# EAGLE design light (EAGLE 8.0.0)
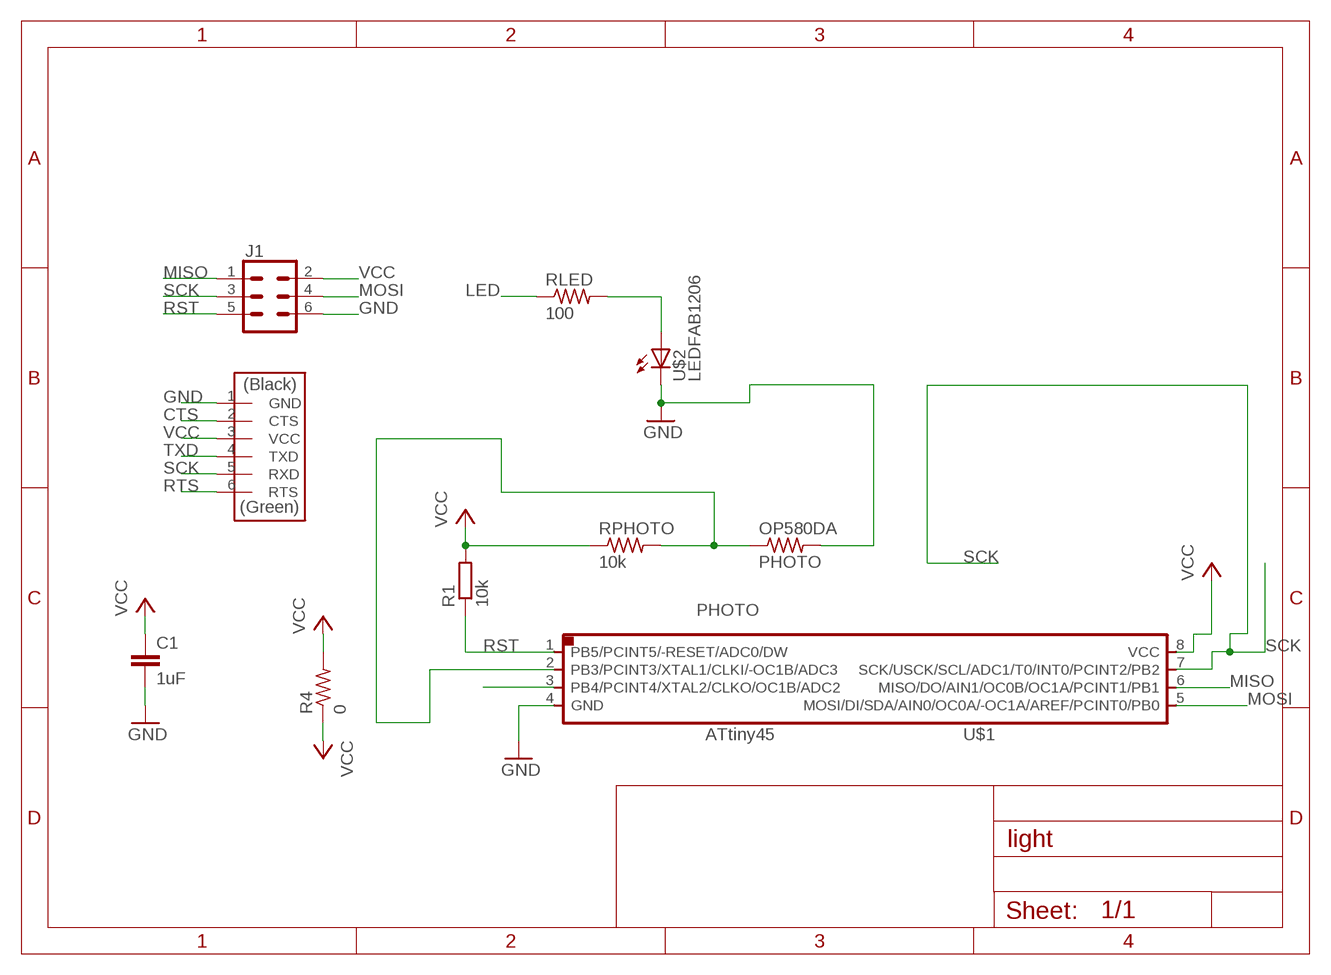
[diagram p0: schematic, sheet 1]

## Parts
C1  1uF  C-EUC1206  [C1206]
J1  CONN_03X2SMT  [2X3_SMT_POSTS]
J2  FTDI-SMD-HEADER  [1X06SMD]
OP580DA  PHOTO  RES-US1206  [R1206]
R1  10k  R-EU_M1206  [M1206]
R4  0  RES-US1206FAB  [R1206FAB]
RLED  100  RES-US1206  [R1206]
RPHOTO  10k  RES-US1206  [R1206]
U$1  ATTINY45SI  [SOIC8]
U$2  LEDFAB1206  [LED1206FAB]

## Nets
CTS: J2.2(CTS)
GND: C1.2 J1.6 J2.1(GND) OP580DA.2 U$1.4(GND) U$2.2(C)
LED: RLED.1 U$1.3(PB4/PCINT4/XTAL2/CLKO/OC1B/ADC2)
MISO: J1.1 U$1.6(MISO/DO/AIN1/OC0B/OC1A/PCINT1/PB1)
MOSI: J1.4 U$1.5(MOSI/DI/SDA/AIN0/OC0A/-OC1A/AREF/PCINT0/PB0)
N$1: RLED.2 U$2.1(A)
PHOTO: OP580DA.1 RPHOTO.2 U$1.2(PB3/PCINT3/XTAL1/CLKI/-OC1B/ADC3)
RST: J1.5 R1.1 U$1.1(PB5/PCINT5/-RESET/ADC0/DW)
RTS: J2.6(RTS)
SCK: J1.3 J2.5(RXD) U$1.7(SCK/USCK/SCL/ADC1/T0/INT0/PCINT2/PB2)
TXD: J2.4(TXD)
VCC: C1.1 J1.2 J2.3(VCC) R1.2 R4.1 R4.2 RPHOTO.1 U$1.8(VCC)

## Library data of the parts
C1 = rcl:C-EU: CAPACITOR, European symbol
J1 = SparkFun-Connectors:CONN_03X2: Multi connection point. Often used as Generic Header-pin footprint for 0.1 inch spaced/style header connections You can populate with any combo of single row headers, but if you'd like an exact match, check these: Header - 2x3 (Male, 0.1") (PRT-12807) Header - 2x3 (Female, 0.1") (PRT-13010) 2x3 Pin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; PROD_ID: CONN-11415
J2 = fab:FTDI-SMD-HEADER
OP580DA R4 RLED RPHOTO = fab:RES-US: Resistor (US Symbol)
R1 = rcl:R-EU_: RESISTOR, European symbol
U$1 = fab:ATTINY45
U$2 = fab:LED: LED

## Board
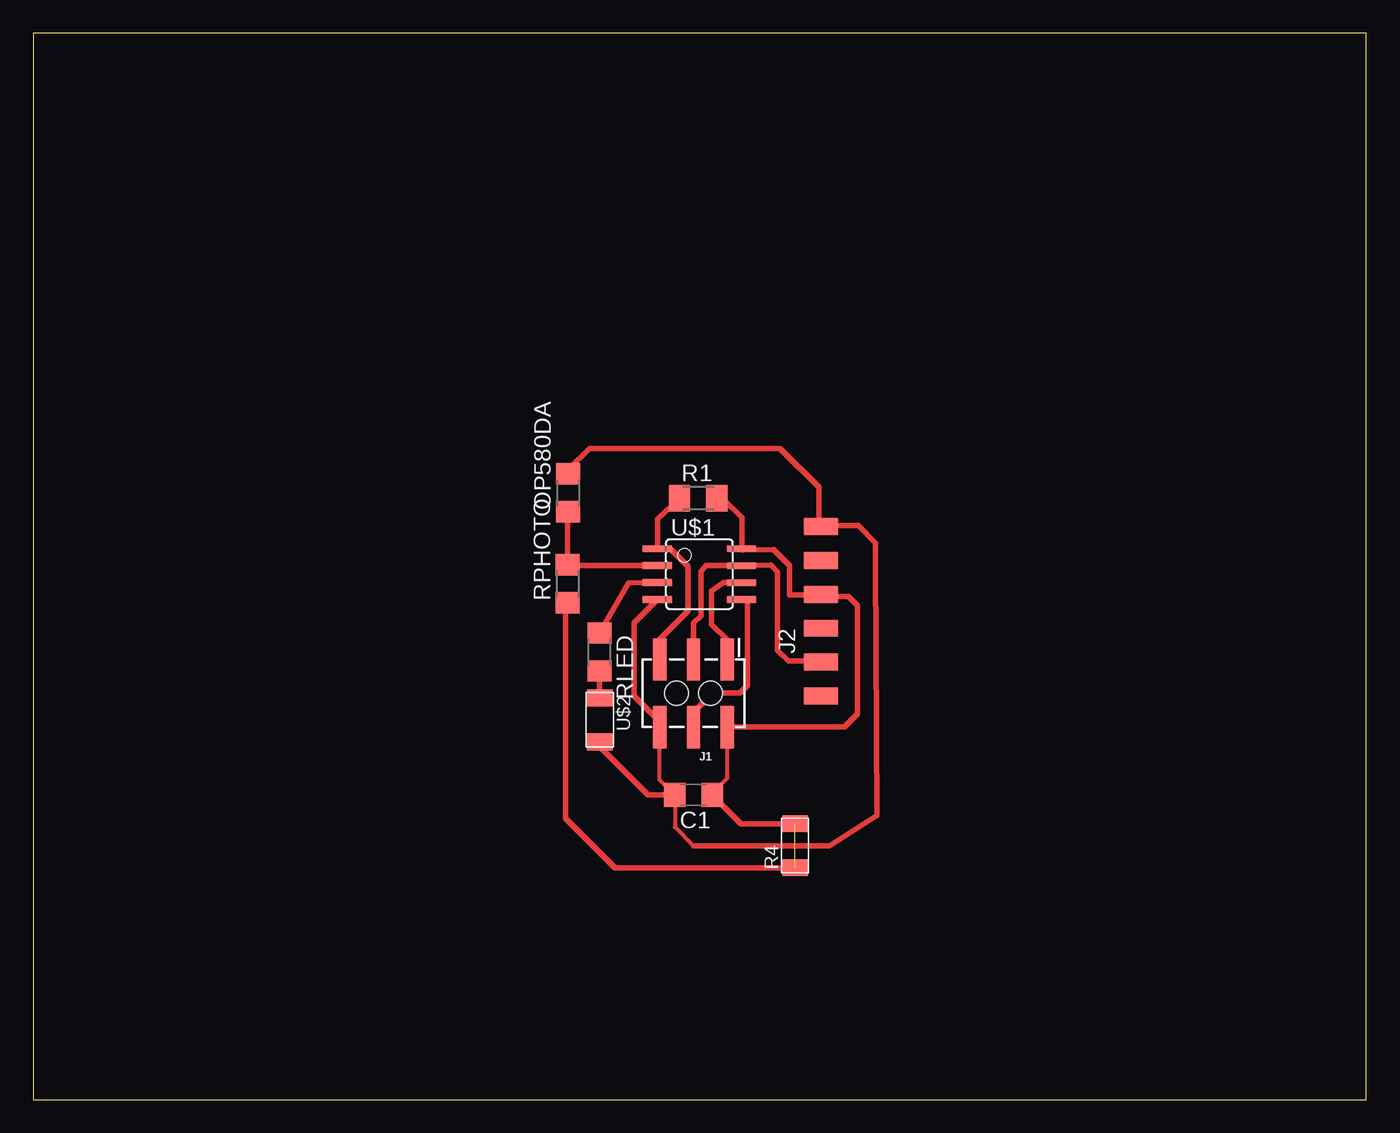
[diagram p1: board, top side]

Size 100 x 80 mm. Coordinates in mm from the lower left corner, seen from the top.
Outline: 0,0 100,0 100,80 0,80 0,0
Copper layers (1*16): Top 0.035mm / dielectric 1.5mm / Bottom 0.035mm
Design rules "default *": minimum track width 12mil, minimum drill 16mil, track to track 16mil, track to pad 16mil, pad to pad 16mil, via to via 16mil, smd to smd 16mil, copper to edge 16mil, drill to drill 16mil, minimum pad ring 10mil, minimum via ring 8mil, stop-mask expansion 4mil, vias tented up to drill 0mil, thermal gap 10mil

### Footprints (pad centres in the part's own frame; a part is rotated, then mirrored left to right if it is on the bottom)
C1206 = smd 1.6 x 1.8: 1 -1.4,0; 2 1.4,0
2X3_SMT_POSTS = smd 1 x 3.17: 1 -2.54,-2.54; 2 -2.54,2.54; 3 0,-2.54; 4 0,2.54; 5 2.54,-2.54; 6 2.54,2.54 | hole 1.8: -1.27,0; 1.27,0
1X06SMD = smd 2.54 x 1.27: 1 0,6.35; 2 0,3.81; 3 0,1.27; 4 0,-1.27; 5 0,-3.81; 6 0,-6.35
R1206 = smd 1.6 x 1.803: 1 -1.422,0; 2 1.422,0
M1206 = smd 1.6 x 2: 1 -1.4,0; 2 1.4,0
R1206FAB = smd 1.27 x 1.905: 1 -1.651,0; 2 1.651,0
SOIC8 = smd 0.5 x 2.2: 1 -1.905,-3.154; 2 -0.645,-3.154; 3 0.625,-3.154; 4 1.895,-3.154; 5 1.905,3.154; 6 0.635,3.154; 7 -0.635,3.154; 8 -1.905,3.154
LED1206FAB = smd 1.27 x 1.905: 1 -1.651,0; 2 1.651,0

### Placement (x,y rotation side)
C1  49.53,22.86 180 top
J1  49.53,30.48 180 top
J2  59.1,36.63 0 top
OP580DA  40.12,45.52 90 top
R1  49.89,45.1 0 top
R4  57.15,19.05 90 top
RLED  42.49,33.58 270 top
RPHOTO  40.09,38.7 90 top
U$1  49.97,39.42 270 top
U$2  42.5,28.49 270 top

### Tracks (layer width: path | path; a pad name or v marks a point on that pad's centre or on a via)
GND
  Top 0.305: J1.6 46.99,24 C1.2 48.13,20.45 49.53,19.05
  Top 0.406: J1.6 46.99,28.35 45.06,30.28 45.06,35.77 U$1.4 | 49.53,19.05 59.73,19.05 63.3,21.32 63.18,40.19 63.18,41.76 61.89,43.06 59.18,43.06 J2.1 58.92,43.16 58.92,45.94 56.03,48.84 45.02,48.84 45,48.85 41.72,48.85 40.12,47.26 OP580DA.2 | U$2.2 42.5,26.48 46.11,22.87 C1.2
LED
  Top 0.406: U$1.3 44.67,38.77 RLED.1
MISO
  Top 0.406: J1.1 52.07,34.47 50.9,35.64 50.9,38.16 51.79,38.78 53.14,38.78 U$1.6
MOSI
  Top 0.406: J1.4 49.53,29.06 50.99,30.51 53.02,30.51 53.59,31.08 53.59,36.97 | 53.59,37.35 53.59,36.97 | 53.59,37.35 53.72,37.48 53.59,37.35 | 53.59,36.97 53.59,37.35 | U$1.5 53.44,37.51 53.59,37.35
N$1
  Top 0.406: RLED.2 42.49,30.16 U$2.1
PHOTO
  Top 0.406: OP580DA.1 40.09,43.71 RPHOTO.2 40.15,40.06 U$1.2 46.19,40.11
RST
  Top 0.305: 46.99,34.29 J1.5
  Top 0.406: J1.5 46.99,34.53 49.12,36.66 49.11,40.01 47.81,41.31 47.13,41.29 | 47.13,41.29 46.3,41.26 | R1.1 46.82,43.56 U$1.1 47.09,41.32 47.13,41.29
SCK
  Top 0.406: J1.3 49.53,35.77 50.08,36.28 50.08,39.63 50.48,40.07 53.11,40.07 U$1.7 55.33,40.11 55.84,39.6 55.84,34.69 | 55.84,34.69 55.84,34.48 | 55.84,34.69 55.84,33.7 56.66,32.89 59.03,32.89 J2.5
VCC  (1 unrouted)
  Top 0.305: C1.1 50.93,22.99 52.07,24.13 J1.2
  Top 0.406: C1.1 53.09,20.7 R4.2 | R1.2 51.71,45.1 53.16,43.65 53.16,41.36 U$1.8 53.22,41.23 55.54,41.28 56.75,40.08 56.75,37.87 58.93,37.87 J2.3 59.27,37.73 61.17,37.73 61.82,37.08 61.82,28.91 60.84,27.94 J1.2 | RPHOTO.1 39.92,37.01 39.92,21.11 43.63,17.4 R4.1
